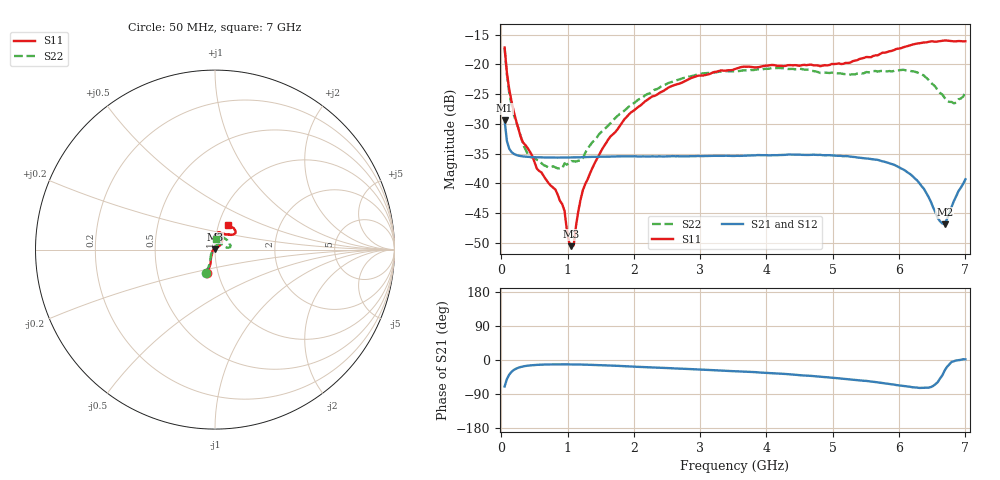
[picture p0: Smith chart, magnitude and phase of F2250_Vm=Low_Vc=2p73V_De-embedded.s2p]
! Integrated Device Technology
! Corporate Headquarters
! 6024 Silver Creek Valley Road
! San Jose, CA 95138  USA
! Phone:  1-408-284-8200
! Toll Free:  1-800-223-1366
! Webpage:  http://www.idt.com/
! Timing and RF Division
! 515 Groton Road, Suite 102
! Westford, MA 01886-6024
! Device:  F2250
! Description: Voltage Variable RF Attenuator
! Frequency:  50.0 -  6000.00 MHz
! Package:  3x3 mm Thin QFN Plastic Package: 16 pin
! Ports:  2 RF, 3 DC
!  Pin  1  = GND
!  Pin  2  = NC
!  Pin  3  = RF1  = Port 1
!  Pin  4  = NC
!  Pin  5  = GND
!  Pin  6  = GND
!  Pin  7  = GND
!  Pin  8  = GND
!  Pin  9  = NC
!  Pin 10  = RF2  = Port 2
!  Pin 11  = NC
!  Pin 12  = GND
!  Pin 13  = GND
!  Pin 14  = VCNTRL
!  Pin 15  = VDD
!  Pin 16  = VMODE
! Vcntrl:  2.730 Volts
! Vmode:  +0.000 Volts
! Vdd:  +3.30  Volts
! Current:  1.174 mA
! Data:  The device was measured on a the F2250 evaluation board which has
!  individual transmission lines to the RF pins.  Data was collected
!  using a calibrated network analyzer.  The evaluation board was
!  de-embedded using a TRL calibration technique.
!  The reference plane is the edge of the package pin.
! Misc:  SN 10
!  Action Tracker AT0258
! Date Measured:  2014-11-26
! Date:  2015-10-15  MJV
! Note:
!  Integrated Device Technology supplies this data as a sample of measured
!  data at the package pin for this product.  Your particular data for this
!  product may vary.
!  Data was taken at 25 degrees C.
!  Integrated Device Technology reserves the right to change this data at anytime.
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# GHz S dB R 50
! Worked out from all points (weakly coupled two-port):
!   201 points, 50 MHz to 7 GHz, reference 50 ohm
!   highest |S21| = -29.41 dB at 50 MHz (marker M1); lowest = -46.9 dB at 6.687 GHz (marker M2)
!   lowest |S11| = -50.6 dB at 1.058 GHz (marker M3), VSWR 1.01, Z = 49.8 + j0.247 ohm
!   |S11| at or under -10 dB: start of sweep to end of sweep
!   |S22| runs from -37.5 to -17.3 dB; largest |S21 - S12| = 5.3e-05
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0.05  -17.18 -108.6  -29.41 -69.8  -29.41 -69.8  -17.27 -111.0
0.08475  -21.45 -107.5  -32.92 -50.3  -32.91 -50.4  -21.75 -110.2
0.15425  -26.23 -116.6  -34.76 -31.1  -34.76 -31.1  -26.81 -122.4
0.29325  -32.22 -127.8  -35.43 -18.5  -35.43 -18.5  -32.09 -137.4
0.3975  -34.08 -141.7  -35.56 -15.0  -35.56 -15.0  -35.05 -160.4
0.91875  -43.51 157.9  -35.68 -11.5  -35.68 -11.5  -37.53 133.5
0.9535  -44.64 170.1  -35.68 -11.5  -35.68 -11.5  -36.66 131.1
1.023  -49.94 143.4  -35.68 -11.6  -35.67 -11.6  -36.64 115.9
1.05775  -50.58 123.2  -35.66 -11.6  -35.67 -11.6  -36.28 110.7
1.0925  -50.44 90.1  -35.66 -11.7  -35.65 -11.7  -36.30 106.5
1.162  -44.67 56.7  -35.64 -11.9  -35.64 -11.9  -36.22 95.5
1.2315  -41.13 44.2  -35.61 -12.1  -35.61 -12.1  -35.79 85.8
1.6485  -32.11 41.9  -35.52 -14.6  -35.52 -14.6  -29.87 64.5
1.96125  -28.05 42.2  -35.46 -17.2  -35.47 -17.2  -26.81 56.8
2.37825  -24.87 47.3  -35.48 -20.3  -35.48 -20.3  -23.99 56.8
3.525  -20.80 72.5  -35.41 -29.5  -35.40 -29.5  -21.19 74.7
4.7065  -20.17 72.3  -35.20 -42.5  -35.20 -42.6  -21.14 72.3
5.85325  -17.81 40.5  -36.64 -63.3  -36.63 -63.4  -21.14 23.0
6.27025  -16.50 40.1  -39.50 -72.7  -39.50 -72.7  -21.36 9.6
6.68725  -15.99 48.8  -46.87 -27.6  -46.81 -27.2  -25.65 28.5
6.861  -16.13 55.1  -42.19 -1.3  -42.15 -1.4  -26.46 58.0
7  -16.13 63.2  -39.34 1.9  -39.31 1.7  -24.63 83.2
